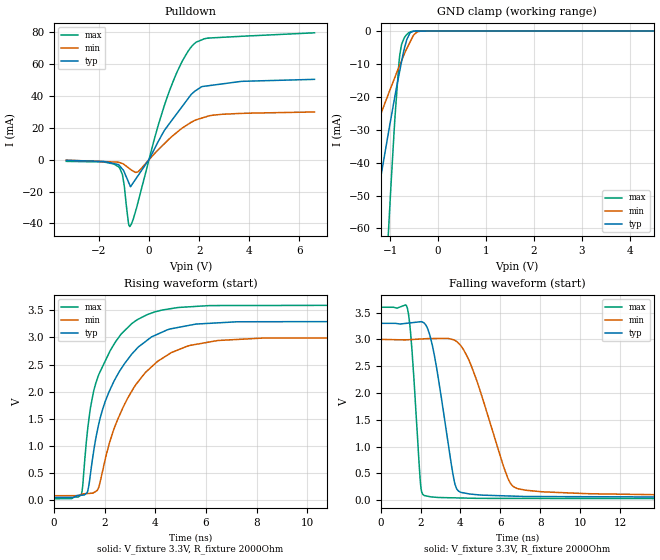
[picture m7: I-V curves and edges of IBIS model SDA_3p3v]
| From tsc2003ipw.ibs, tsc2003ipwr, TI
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|   SDA_3p3v
[Model]   SDA_3p3v
Model_type   I/O_open_drain
Polarity   Non-Inverting
Enable   Active-High
Vinl = 0.99
Vinh = 2.31
Vmeas = 1.65
Vref = 1.65
Cref = 1pF
Rref = 50
|   typ   min   max
C_comp   0.526pF   0.447pF   0.563pF
[Voltage Range]   3.3   3   3.6
[Temperature Range]   27   85   -40
[Pullup Reference]   3.3   3   3.6
[Pulldown Reference]   0   0   0
[Power Clamp Reference]   3.3   3   3.6
[GND Clamp Reference]   0   0   0
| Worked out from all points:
|   slope of the pulldown table from 0 to 0.495 V, typ, clamps not added: 33.2 ohm
|   GND clamp passes 1 mA (typ) near -0.60 V on its own axis
|   falling waveform, V_fixture 3.3V, R_fixture 2000Ohm: 20-80 % time 813ps typ, 1.49ns min, 366ps max; typ from 3.3 V to 0.05 V
|   rising waveform, V_fixture 3.3V, R_fixture 2000Ohm: 20-80 % time 1.5ns typ, 1.77ns min, 1.17ns max; typ from 0.049 V to 3.3 V
[Pulldown]
|   Voltage   I(typ)   I(min)   I(max)
-3.3V     -414uA     -279.7uA   -1.055mA
-1.207V   -3.189mA   -1.625mA   -4.547mA
-1.059V   -5.935mA   -2.431mA   -9.324mA
-817.3mV  -14.04mA   -5.105mA   -40.03mA
-764.5mV  -15.98mA   -5.741mA   -42mA
-443.3mV  -10.18mA   -7.695mA   -27.06mA
649.1mV   19.16mA    10.58mA    35.75mA
1.336V    33.67mA    19.93mA    62.15mA
1.771V    42.22mA    24.2mA     72.34mA
2.323V    46.34mA    27.17mA    76.26mA
3.687V    49.19mA    29.07mA    77.47mA
6.6V      50.44mA    29.96mA    79.66mA
[GND Clamp]
|   Voltage   I(typ)   I(min)   I(max)
-3.3V     -229.6mA   -108.6mA   -718.4mA
-2.204V   -132.3mA   -64.84mA   -397.2mA
-2.013V   -115.5mA   -57.25mA   -341.2mA
-1.405V   -62.21mA   -33.28mA   -164.3mA
-1.059V   -32.6mA    -19.89mA   -66.48mA
-1.023V   -29.61mA   -18.53mA   -57.01mA
-905.6mV  -20.01mA   -14.13mA   -26.91mA
-799.7mV  -11.92mA   -10.26mA   -7.047mA
-711.3mV  -5.611mA   -7.139mA   -2.129mA
-572.4mV  -396.2uA   -2.906mA   -196.3uA
-353.4mV  -25.4uA    -20.38uA   -488.9nA
6.6V      0A         0A         0A
[POWER Clamp]
|   Voltage   I(typ)   I(min)   I(max)
-3.3V     0A         0A         0A
0V        0A         0A         0A
6.6V      0A         0A         0A
[Ramp]
R_load = 2000
|   typ   min   max
dV/dt_r   1.95079/1.4917e-009   1.75119/1.75844e-009   2.14396/1.16525e-009
dV/dt_f   1.95003/8.11338e-010   1.74653/1.48888e-009   2.14394/3.6543e-010
[Falling Waveform]
V_fixture = 3.3V
V_fixture_min = 3V
V_fixture_max = 3.6V
R_fixture = 2000Ohm
C_fixture = 0F
|   Time   V(typ)   V(min)   V(max)
0s        3.3V       3V         3.6V
1.339ns   3.302V     2.993V     3.58V
1.559ns   3.311V     2.997V     2.842V
1.994ns   3.33V      3.007V     318.1mV
2.171ns   3.308V     3.011V     89.33mV
2.685ns   2.714V     3.016V     55.71mV
3.685ns   360.3mV    2.989V     42.65mV
3.992ns   149.5mV    2.894V     40.18mV
6.846ns   72.34mV    216.7mV    32.23mV
20.74ns   49.96mV    89.11mV    26.77mV
[Rising Waveform]
V_fixture = 3.3V
V_fixture_min = 3V
V_fixture_max = 3.6V
R_fixture = 2000Ohm
C_fixture = 0F
|   Time   V(typ)   V(min)   V(max)
0s        48.68mV    81.33mV    26.73mV
1.088ns   90.87mV    104.2mV    111.9mV
1.339ns   169mV      122.4mV    1.329V
1.709ns   1.265V     178mV      2.231V
2.018ns   1.808V     734.4mV    2.557V
2.495ns   2.298V     1.463V     2.96V
3.691ns   2.952V     2.389V     3.423V
4.637ns   3.161V     2.722V     3.533V
6.465ns   3.269V     2.944V     3.588V
20.74ns   3.3V       3V         3.6V
